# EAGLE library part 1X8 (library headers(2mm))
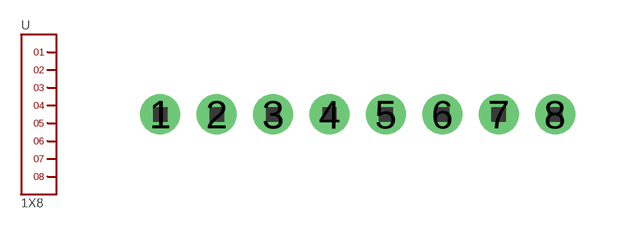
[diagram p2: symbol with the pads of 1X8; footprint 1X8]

Designator prefix -

## 1X8  [1X8]
1  1
2  2
3  3
4  4
5  5
6  6
7  7
8  8

## Footprint 1X8 (pad centres in mm)
drill 0.8 pad 1.422: 1 -7,0; 2 -5,0; 3 -3,0; 4 -1,0; 5 1,0; 6 3,0; 7 5,0; 8 7,0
